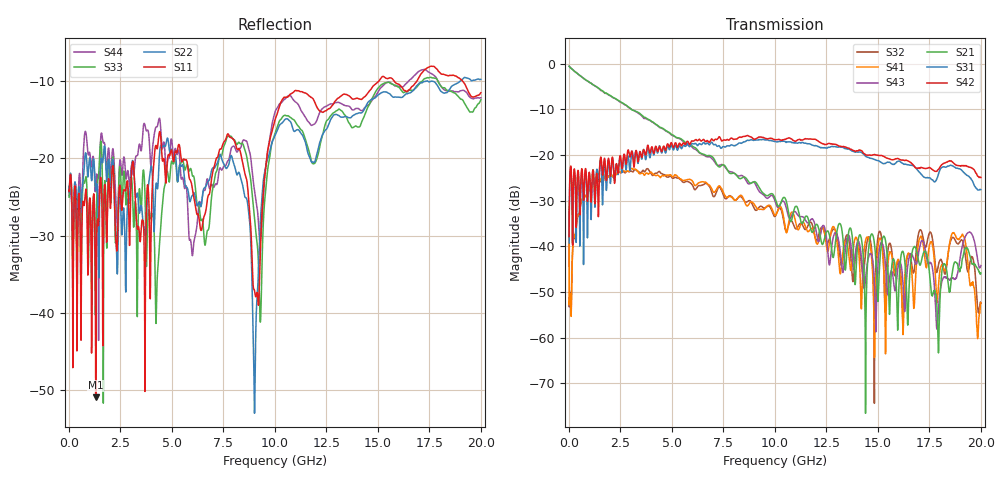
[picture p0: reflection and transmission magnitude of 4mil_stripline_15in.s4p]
! FILE: C:\Archive\Backplane\4-mil striplines\4mil_stripline_15in.s4p
! SMA ->1inch 21mil width microstrip -> 15 inch 4-mil width stripline -> 1 inch 21mil width microstrip -> SMA
! Port 1 -> Port 2, Port 3 -> Port 4
! 10/8/08
# MHz S DB R 50.00
! FREQ  S11  S12  S13  S14
!  S21  S22  S23  S24
!  S31  S32  S33  S34
!  S41  S42  S43  S44
!  DB  ANG  DB  ANG  DB  ANG  DB  ANG
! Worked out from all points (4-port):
!   2000 points, 10 MHz to 20 GHz, reference 50 ohm
!   strongest paths, dB at 10 MHz, 5.01 GHz, 10.01 GHz, 15.01 GHz, 20 GHz:
!     S42: -37.9, -17.7, -16.6, -20.1, -24.9
!     S31: -39.3, -18.2, -17.1, -21.2, -27.6
!     S21: -0.5, -15.6, -29.5, -51.7, -45.8
!     S43: -0.5, -15.7, -30.1, -43.6, -44.2
!     S41: -32.6, -24.7, -33.2, -39.9, -52.4
!     S32: -31.2, -25.0, -33.4, -37.8, -52.4
!   lowest |S11| = -50.9 dB at 1.3 GHz (marker M1), VSWR 1.01, Z = 49.8 + j0.202 ohm
!   |S11| at or under -10 dB: start of sweep to 15.06 GHz; 15.79 GHz to 16.9 GHz (1.113 GHz wide, 6.81 % of centre); 19.1 GHz to end of sweep
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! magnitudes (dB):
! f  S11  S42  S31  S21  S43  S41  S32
! 10 MHz  -24.2  -37.9  -39.3  -0.5  -0.5  -32.6  -31.2
! 1.3 GHz  -50.9  -26.7  -26.7  -4.9  -4.9  -25.7  -25.6
! 7.91 GHz  -17.4  -16.3  -17.8  -24.0  -23.7  -29.3  -29.1
! 9.02 GHz  -37.2  -16.5  -16.7  -25.8  -26.1  -30.9  -31.9
! 10.28 GHz  -12.8  -16.7  -17.0  -30.5  -30.6  -31.3  -31.8
! 17.88 GHz  -8.5  -23.4  -25.0  -54.6  -58.1  -52.3  -45.5
! 20 GHz  -11.5  -24.9  -27.6  -45.8  -44.2  -52.4  -52.4
